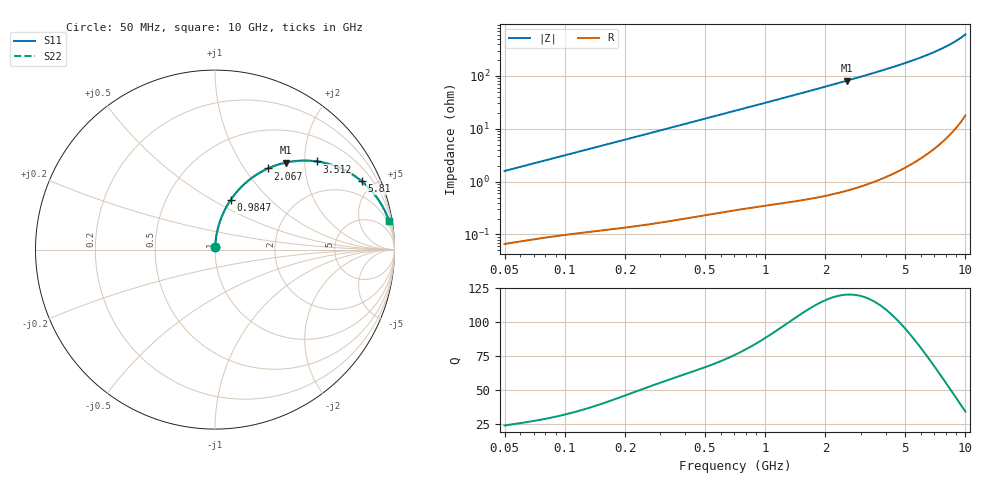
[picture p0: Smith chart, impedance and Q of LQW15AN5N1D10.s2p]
!Murata Part Number: LQW15AN5N1D10
!These Parameters are Measured in Series Mode Connection
!  o--[Z]--o
!Port1  Port2
!  o-------o
!Freq. Start=50[MHz] Stop=10[GHz], 401[Steps]
# Hz S RI R 50
!Freq.(Hz)	S 11(Real)	S 11(Imag)	S 21(Real)	S 21(Imag)	S 12(Real)	S 12(Imag)	S 22(Real)	S 22(Imag)
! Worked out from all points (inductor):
!   401 points, 50 MHz to 10 GHz, reference 50 ohm
!   read as one part in series: L = 5.03 nH near 51.34 MHz
!   highest Q = 120 at 2.556 GHz (marker M1), where L = 5.03 nH
!   S11 on the Smith chart (normalised r, x): 50 MHz: 1.00, +0.03; 984.7 MHz: 1.01, +0.61; 2.067 GHz: 1.01, +1.29; 3.512 GHz: 1.02, +2.29; 5.81 GHz: 1.05, +4.26; 10 GHz: 1, +12
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5e7  0.000913 0.0158  0.9991 -0.0158  0.9991 -0.0158  0.000913 0.0158
1.214486e8  0.00251 0.0378  0.9975 -0.0378  0.9975 -0.0378  0.00251 0.0378
1.956524e8  0.005 0.0604  0.995 -0.0604  0.995 -0.0604  0.005 0.0604
2.949953e8  0.00989 0.0903  0.9901 -0.0903  0.9901 -0.0903  0.00989 0.0903
4.628099e8  0.0221 0.1394  0.9779 -0.1394  0.9779 -0.1394  0.0221 0.1394
7.071068e8  0.0478 0.2069  0.9522 -0.2069  0.9522 -0.2069  0.0478 0.2069
9.846897e8  0.087 0.2761  0.913 -0.2761  0.913 -0.2761  0.087 0.2761
1.31782e9  0.1447 0.3468  0.8553 -0.3468  0.8553 -0.3468  0.1447 0.3468
1.504464e9  0.1806 0.38  0.8194 -0.38  0.8194 -0.38  0.1806 0.38
1.717543e9  0.2235 0.4122  0.7765 -0.4122  0.7765 -0.4122  0.2235 0.4122
2.067491e9  0.2961 0.4523  0.7039 -0.4523  0.7039 -0.4523  0.2961 0.4523
2.555552e9  0.3955 0.4848  0.6045 -0.4848  0.6045 -0.4848  0.3955 0.4848
2.99582e9  0.479 0.4954  0.521 -0.4954  0.521 -0.4954  0.479 0.4954
3.511936e9  0.566 0.4913  0.434 -0.4913  0.434 -0.4913  0.566 0.4913
4.171863e9  0.6592 0.4693  0.3408 -0.4693  0.3408 -0.4693  0.6592 0.4693
4.890587e9  0.7397 0.4337  0.2603 -0.4337  0.2603 -0.4337  0.7397 0.4337
5.809576e9  0.8167 0.381  0.1833 -0.381  0.1833 -0.381  0.8167 0.381
6.810442e9  0.876 0.3225  0.124 -0.3225  0.124 -0.3225  0.876 0.3225
7.775012e9  0.9161 0.2688  0.0839 -0.2688  0.0839 -0.2688  0.9161 0.2688
8.759398e9  0.9449 0.2178  0.0551 -0.2178  0.0551 -0.2178  0.9449 0.2178
9.738562e9  0.9648 0.1711  0.0352 -0.1711  0.0352 -0.1711  0.9648 0.1711
1e10  0.969 0.1593  0.031 -0.1593  0.031 -0.1593  0.969 0.1593
